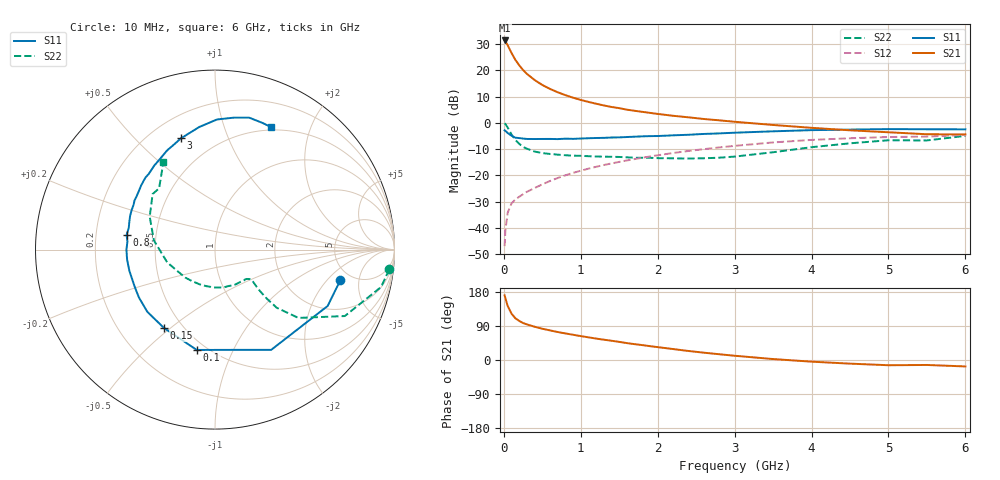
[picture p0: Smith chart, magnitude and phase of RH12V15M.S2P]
! SIEMENS Small Signal Semiconductors
! BFR106
! Si NPN RF Bipolar Junction Transistor in SOT23
! VCE = 12 V  IC = 15 mA
! Common Emitter S-Parameters:  August  1996
# GHz  S  MA  R  50
!  f  S11  S21  S12  S22
! GHz  MAG  ANG  MAG  ANG  MAG  ANG  MAG  ANG
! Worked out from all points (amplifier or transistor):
!   36 points, 10 MHz to 6 GHz, reference 50 ohm
!   highest |S21| = 31.3 dB at 10 MHz (marker M1)
!   |S21| within 3 dB of that: start of sweep to 70.11 MHz
!   unconditionally stable (mu >= 1): 432.8 MHz to 2.076 GHz
!   at 250 MHz: K = 0.80, MSG = 23.6 dB, |S12| = -27.2 dB
!   at 1.4 GHz: K = 1.08, MAG = 9.0 dB, |S12| = -15.4 dB
!   at 6 GHz: K = 0.99, MSG = 0.1 dB, |S12| = -4.6 dB
!   S11 on the Smith chart (normalised r, x): 10 MHz: 4.05, -2.84; 100 MHz: 0.44, -0.73; 150 MHz: 0.40, -0.47; 800 MHz: 0.34, +0.07; 3 GHz: 0.32, +0.69; 6 GHz: 0.47, +1.46
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0.01  0.7193 -13.6  36.87 170.5  0.0045 83.0  0.977 -6.5
0.02  0.7018 -26.6  35.59 163.1  0.009 79.8  0.9485 -12.7
0.05  0.6403 -60.7  29.91 142.5  0.0195 63.4  0.8126 -27.1
0.1  0.5682 -100.3  21.32 122.3  0.0293 54.5  0.6009 -39.3
0.15  0.5209 -123.2  15.75 110.1  0.0349 50.9  0.4723 -43.3
0.2  0.5122 -137.4  12.43 103.1  0.0392 52.1  0.3989 -43.4
0.25  0.5009 -147.8  10.1 97.6  0.0438 53.3  0.3489 -42.8
0.3  0.493 -155.1  8.527 93.9  0.0487 56.0  0.3214 -42.2
0.4  0.4915 -166.0  6.52 87.8  0.0574 59.1  0.2839 -40.5
0.5  0.4929 -173.3  5.245 82.5  0.0675 61.3  0.2652 -39.5
0.6  0.4936 -179.9  4.414 78.1  0.0782 63.1  0.2559 -40.1
0.7  0.4898 174.7  3.814 73.9  0.0891 64.2  0.248 -41.3
0.8  0.4995 170.6  3.36 70.1  0.1003 64.5  0.2416 -42.6
1.1  0.5089 158.3  2.499 59.8  0.1342 64.7  0.2317 -49.4
1.3  0.5173 151.4  2.14 53.6  0.1574 63.9  0.2268 -54.9
1.6  0.5365 141.9  1.778 44.6  0.1925 61.9  0.2205 -65.4
2.2  0.5775 125.9  1.361 28.9  0.2663 56.0  0.2111 -91.2
3  0.6483 107.0  1.047 11.2  0.3643 45.5  0.2277 -136.8
3.5  0.6888 97.3  0.91 2.5  0.4234 37.9  0.2754 -164.9
4.5  0.7429 81.8  0.72 -9.6  0.5084 21.5  0.4072 153.3
5.5  0.7537 69.4  0.606 -13.1  0.5465 9.8  0.4619 132.4
6  0.7507 65.3  0.602 -17.0  0.588 2.0  0.565 120.6
